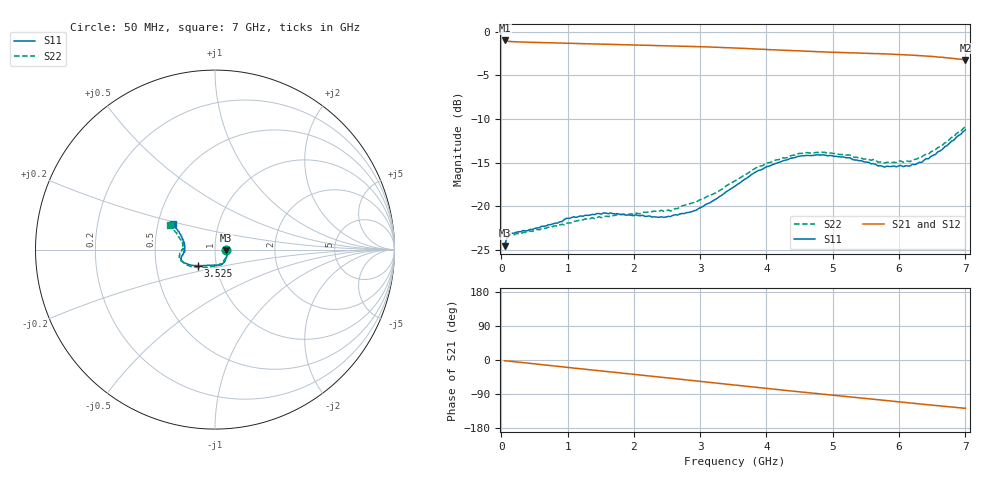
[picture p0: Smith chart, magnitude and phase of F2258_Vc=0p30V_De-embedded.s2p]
! Integrated Device Technology
! Corporate Headquarters
! 6024 Silver Creek Valley Road
! San Jose, CA 95138  USA
! Phone:  1-408-284-8200
! Toll Free:  1-800-223-1366
! Webpage:  http://www.idt.com/
! Timing and RF Division
! 515 Groton Road, Suite 102
! Westford, MA 01886-6024
! Device:  F2258
! Description: Voltage Variable RF Attenuator
! Frequency:  50.0 -  6000.00 MHz
! Package:  3x3 mm Thin QFN Plastic Package: 16 pin
! Ports:  2 RF, 2 DC
!  Pin  1  = NC
!  Pin  2  = NC
!  Pin  3  = RF2  = Port 2
!  Pin  4  = GND
!  Pin  5  = Vdd
!  Pin  6  = NC
!  Pin  7  = VCTRL
!  Pin  8  = NC
!  Pin  9  = GND
!  Pin 10  = RF1  = Port 1
!  Pin 11  = NC
!  Pin 12  = NC
!  Pin 13  = NC
!  Pin 14  = NC
!  Pin 15  = NC
!  Pin 16  = NC
! Vcntrl:  0.300 Volts
! Vdd:  +3.300 Volts
! Current:  1.087 mA
! Data:  The device was measured on a the F2258 evaluation board which has
!  individual transmission lines to the RF pins.  Data was collected
!  using a calibrated network analyzer.  The evaluation board was
!  de-embedded using a TRL calibration technique.
!  The reference plane is the edge of the package pin.
! Misc:  SN 10
!  Action Tracker AT0285
! Date Measured:  2014-12-10
! Date:  2016-01-13  MJV
! Note:
!  Integrated Device Technology supplies this data as a sample of measured
!  data at the package pin for this product.  Your particular data for this
!  product may vary.
!  Data was taken at 25 degrees C.
!  Integrated Device Technology reserves the right to change this data at anytime.
!Freq_(GHz)  S11M_(dB)  S11P_(deg)  S21M_(dB)  S21P_(deg)  S12M_(dB)  S12P_(deg)  S22M_(dB)  S22P_(deg)
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# GHz S dB R 50
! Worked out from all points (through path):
!   201 points, 50 MHz to 7 GHz, reference 50 ohm
!   highest |S21| = -0.98 dB at 50 MHz (marker M1); lowest = -3.2 dB at 7 GHz (marker M2)
!   group delay of S21, straight-line fit = 50.5 ps
!   lowest |S11| = -24.5 dB at 50 MHz (marker M3), VSWR 1.13, Z = 56.3 - j0.398 ohm
!   |S11| at or under -10 dB: start of sweep to end of sweep
!   |S22| runs from -24.6 to -10.9 dB; largest |S21 - S12| = 0.00037
!   S11 on the Smith chart (normalised r, x): 50 MHz: 1.13, -0.01; 3.525 GHz: 0.82, -0.15; 7 GHz: 0.60, +0.19
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0.05  -24.54 -3.4  -0.98 -1.9  -0.98 -1.9  -24.61 -3.0
0.08475  -23.58 -5.8  -1.05 -2.5  -1.05 -2.5  -23.67 -5.4
0.15425  -23.10 -9.0  -1.11 -3.6  -1.11 -3.6  -23.30 -9.3
0.71025  -22.14 -36.3  -1.24 -14.1  -1.24 -14.1  -22.42 -38.1
0.98825  -21.40 -49.9  -1.29 -19.3  -1.29 -19.3  -21.95 -54.0
1.2315  -21.17 -58.1  -1.35 -23.8  -1.35 -23.8  -21.59 -63.0
1.6485  -20.79 -69.7  -1.43 -31.4  -1.43 -31.4  -21.11 -76.0
2.37825  -21.29 -90.8  -1.56 -44.8  -1.56 -44.8  -20.59 -93.7
2.552  -21.21 -96.8  -1.59 -48.0  -1.59 -48.0  -20.56 -99.0
2.93425  -20.49 -113.5  -1.68 -55.1  -1.68 -55.1  -19.58 -112.5
3.247  -19.17 -126.1  -1.76 -61.0  -1.76 -61.0  -18.46 -124.7
3.525  -17.72 -136.6  -1.84 -66.2  -1.84 -66.2  -17.11 -135.2
4.0115  -15.46 -150.5  -2.02 -75.2  -2.02 -75.2  -15.05 -150.7
4.46325  -14.32 -159.0  -2.18 -83.4  -2.18 -83.4  -14.01 -161.8
4.7065  -14.18 -162.3  -2.25 -87.7  -2.25 -87.7  -13.90 -166.1
5.2625  -14.46 -169.2  -2.40 -97.4  -2.41 -97.4  -14.15 -174.1
5.6795  -15.39 -176.0  -2.49 -104.6  -2.49 -104.6  -14.96 -179.6
5.85325  -15.46 179.9  -2.54 -107.8  -2.55 -107.8  -14.99 175.8
6.166  -15.40 172.0  -2.65 -113.4  -2.65 -113.4  -14.90 169.9
6.33975  -14.99 165.6  -2.73 -116.5  -2.74 -116.5  -14.37 165.5
6.722  -13.07 153.8  -2.97 -123.1  -2.97 -123.1  -12.66 156.4
7  -11.25 148.3  -3.21 -127.4  -3.22 -127.4  -10.88 151.5
